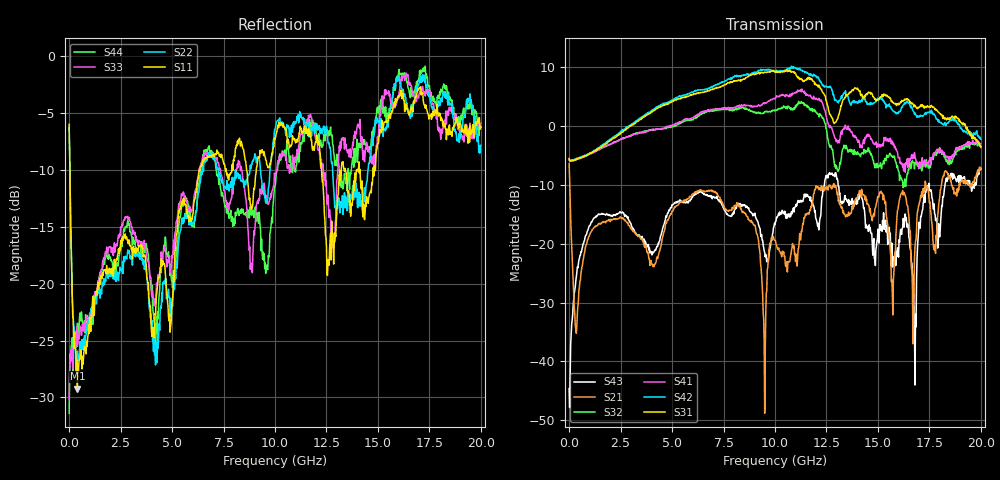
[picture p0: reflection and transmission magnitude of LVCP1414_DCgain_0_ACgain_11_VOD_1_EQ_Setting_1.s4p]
!Agilent Technologies,N5230A,MY46400459,A.07.50.48
!Agilent N5230A: A.07.50.48
!Date: Tuesday, April 17, 2012 18:29:44
!Correction: S11(Full 4 Port(1,2,3,4))
!S12(Full 4 Port(1,2,3,4))
!S13(Full 4 Port(1,2,3,4))
!S14(Full 4 Port(1,2,3,4))
!S21(Full 4 Port(1,2,3,4))
!S22(Full 4 Port(1,2,3,4))
!S23(Full 4 Port(1,2,3,4))
!S24(Full 4 Port(1,2,3,4))
!S31(Full 4 Port(1,2,3,4))
!S32(Full 4 Port(1,2,3,4))
!S33(Full 4 Port(1,2,3,4))
!S34(Full 4 Port(1,2,3,4))
!S41(Full 4 Port(1,2,3,4))
!S42(Full 4 Port(1,2,3,4))
!S43(Full 4 Port(1,2,3,4))
!S44(Full 4 Port(1,2,3,4))
!S4P File: Measurements: <S11,S12,S13,S14>,
!<S21,S22,S23,S24>,
!<S31,S32,S33,S34>,
!<S41,S42,S43,S44>:
# Hz S  dB  R 50
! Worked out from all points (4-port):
!   801 points, 300 kHz to 20 GHz, reference 50 ohm
!   strongest paths, dB at 300 kHz, 5 GHz, 10 GHz, 15 GHz, 20 GHz:
!     S31: -5.5, 4.1, 9.1, 4.4, -3.6
!     S42: -5.8, 4.4, 9.3, 4.6, -2.3
!     S41: -5.6, 0.2, 4.6, -3.2, -3.0
!     S32: -5.7, -0.1, 2.6, -7.1, -3.5
!     S21: -6.4, -14.5, -19.4, -12.0, -7.4
!     S43: -44.6, -13.4, -16.7, -17.5, -7.2
!   lowest |S11| = -29.2 dB at 400.3 MHz (marker M1), VSWR 1.07, Z = 53.3 + j1.38 ohm
!   |S11| at or under -10 dB: 37.72 MHz to 6.322 GHz (6.284 GHz wide, 198 % of centre); 12.26 GHz to 13.22 GHz (954.6 MHz wide, 7.49 % of centre); 14.13 GHz to 14.77 GHz (640.4 MHz wide, 4.43 % of centre)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
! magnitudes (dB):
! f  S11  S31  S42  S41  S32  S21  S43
! 300 kHz  -6.0  -5.5  -5.8  -5.6  -5.7  -6.4  -44.6
! 400.3 MHz  -29.2  -5.5  -5.5  -5.6  -5.6  -31.9  -24.0
! 10 GHz  -7.3  9.1  9.3  4.6  2.6  -19.4  -16.7
! 12.7 GHz  -15.6  1.9  6.6  0.0  -3.6  -10.4  -8.2
! 16.78 GHz  -4.0  3.5  2.0  -4.5  -7.3  -22.5  -34.8
! 17.4 GHz  -4.9  3.5  2.4  -6.4  -6.5  -10.3  -10.2
! 20 GHz  -6.2  -3.6  -2.3  -3.0  -3.5  -7.4  -7.2
